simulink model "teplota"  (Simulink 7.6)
settings: Solver=ode4  StartTime=0.0  StopTime=3000  FixedStep=0.2  RelTol=1e-3
undefined symbols (not defined in the file or in its folder): ABOVE_NORMAL_PRIORITY, COM3, lightbulb

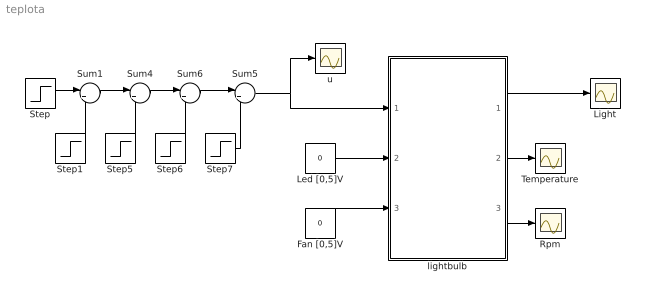
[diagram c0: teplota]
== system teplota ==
  Fan [0,5]V : Constant  Value=0
  Led [0,5]V : Constant  Value=0
  Light : Scope
  Rpm : Scope
  Step : Step  Time=0  After=2  SampleTime=0
  Step1 : Step  Time=600  After=2  SampleTime=0
  Step5 : Step  Time=1200  SampleTime=0
  Step6 : Step  Time=1800  After=-2  SampleTime=0
  Step7 : Step  Time=2400  After=-2  SampleTime=0
  Sum{1,4..6} (4 alike) : Sum  Inputs=|++
  Temperature : Scope
  lightbulb : Subsystem  AncestorBlock=lightbulb/lightbulb
  u : Scope
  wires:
  Fan [0,5]V/1 -> lightbulb/3(fan)
  lightbulb/2(temperature) -> Temperature/1
  lightbulb/3(rpm) -> Rpm/1
  Led [0,5]V/1 -> lightbulb/2(led)
  lightbulb/1(light) -> Light/1
  Step5/1 -> Sum4/2
  Step6/1 -> Sum6/2
  Step7/1 -> Sum5/2
  Sum4/1 -> Sum6/1
  Sum6/1 -> Sum5/1
  Sum1/1 -> Sum4/1
  Step1/1 -> Sum1/2
  Step/1 -> Sum1/1
  Sum5/1 -> lightbulb/1(bulb), u/1

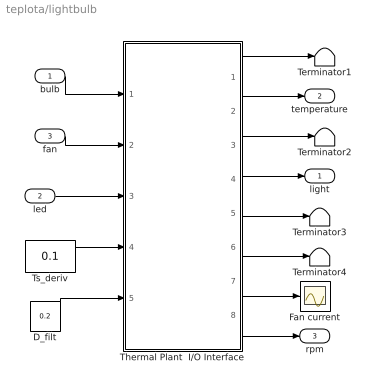
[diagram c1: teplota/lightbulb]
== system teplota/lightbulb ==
  bulb : Inport
  led : Inport  Port=2
  fan : Inport  Port=3
  D_filt : Constant  Value=0.2
  Fan current : Scope
  Terminator{1..4} (4 alike) : Terminator
  Thermal Plant  I/O Interface : Subsystem  mask{Ts=0.2}
      mask prompts: Ts "Sample time (s)"
      mask init:
      | set_param(bdroot,'FixedStep',num2str(Ts));
  Ts_deriv : Constant  Value=0.1
  light : Outport
  temperature : Outport  Port=2
  rpm : Outport  Port=3
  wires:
  bulb/1 -> Thermal Plant  I/O Interface/1(Bulb)
  Thermal Plant  I/O Interface/8(Fan rpm) -> rpm/1
  Thermal Plant  I/O Interface/7(Fan current) -> Fan current/1
  D_filt/1 -> Thermal Plant  I/O Interface/5(D_filt)
  Ts_deriv/1 -> Thermal Plant  I/O Interface/4(Ts_deriv)
  led/1 -> Thermal Plant  I/O Interface/3(LED)
  fan/1 -> Thermal Plant  I/O Interface/2(Fan)
  Thermal Plant  I/O Interface/1(Ambient temperature) -> Terminator1/1
  Thermal Plant  I/O Interface/6(Derivative  of light intensity) -> Terminator4/1
  Thermal Plant  I/O Interface/5(Filtered light intensity) -> Terminator3/1
  Thermal Plant  I/O Interface/4(Light intensity) -> light/1
  Thermal Plant  I/O Interface/2(Temperature) -> temperature/1
  Thermal Plant  I/O Interface/3(Filtered temperature) -> Terminator2/1

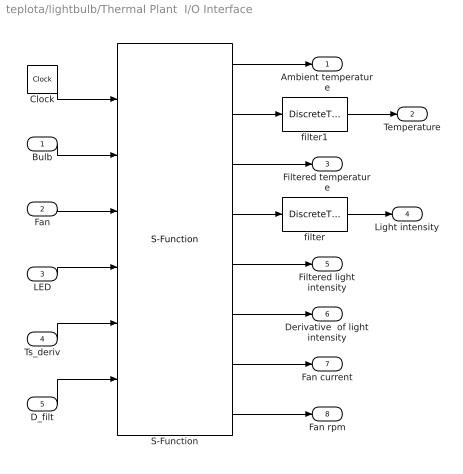
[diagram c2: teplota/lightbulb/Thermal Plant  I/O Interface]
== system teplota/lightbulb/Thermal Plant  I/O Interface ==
  Bulb : Inport
  Fan : Inport  Port=2
  LED : Inport  Port=3
  Ts_deriv : Inport  Port=4
  D_filt : Inport  Port=5
  Clock : Clock
  S-Function : S-Function  Priority=1  FunctionName=udaq28LT_v1R13  Parameters=com_port, Ts, events_ot, rd_timeout, matlab_prior, warning, printout  EnableBusSupport=off  mask(uDAQ28/LT Communication Interface){com_port=COM3, Ts=Ts, events_ot=1, rd_timeout=Ts/2*1000, matlab_prior=ABOVE_NORMAL_PRIORITY, warning=on, printout=off}
      mask prompts: com_port "Serial port:"; Ts "Sample time (sec):"; events_ot "Sampling delayed (%):"; rd_timeout "Read timeout (msec, lower than sample time):"; matlab_prior "Matlab priority"; warning "Warning if delayed (error if unchecked)"; printout "Detailed timing and timeout  printout"
      mask help: (c) 2006 Martin Kamensky Serial port - USB serial port number assigned to uDAQ28/LT system Sampling time (sec) - the lowest working value in Windows is about 0.04 - 0.05 s Sample delayed (%) - number of events (percentually) when simulink loop can take more than time determined by sample time Read timeout (msec) - timeout for reading data from the port (the lowest working value is about 25 ms) Matlab priority : NORMAL_PRIORITY - priority of common Windows application ABOVE_NORMAL_PRIORITY - recommended - higher priority than common Windows application priority HIGH_PRIORITY - recommended - hig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
      mask init:
      | %set_param(bdroot,'FixedStep',get_param(gcb,'Ts'));
      | set_param(bdroot,'Solver','ode4');
  filter : DiscreteTransferFcn  Numerator=0.6  Denominator=[1 -0.4]  SampleTime=Ts
  filter1 : DiscreteTransferFcn  Numerator=0.6  Denominator=[1 -0.4]  SampleTime=Ts
  Ambient temperature : Outport
  Temperature : Outport  Port=2
  Filtered temperature : Outport  Port=3
  Light intensity : Outport  Port=4
  Filtered light intensity : Outport  Port=5
  Derivative  of light intensity : Outport  Port=6
  Fan current : Outport  Port=7
  Fan rpm : Outport  Port=8
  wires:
  S-Function/8 -> Fan rpm/1
  S-Function/7 -> Fan current/1
  S-Function/6 -> Derivative  of light intensity/1
  S-Function/5 -> Filtered light intensity/1
  S-Function/4 -> filter/1
  S-Function/3 -> Filtered temperature/1
  S-Function/2 -> filter1/1
  S-Function/1 -> Ambient temperature/1
  D_filt/1 -> S-Function/6
  Ts_deriv/1 -> S-Function/5
  LED/1 -> S-Function/4
  Fan/1 -> S-Function/3
  Bulb/1 -> S-Function/2
  Clock/1 -> S-Function/1
  filter1/1 -> Temperature/1
  filter/1 -> Light intensity/1
